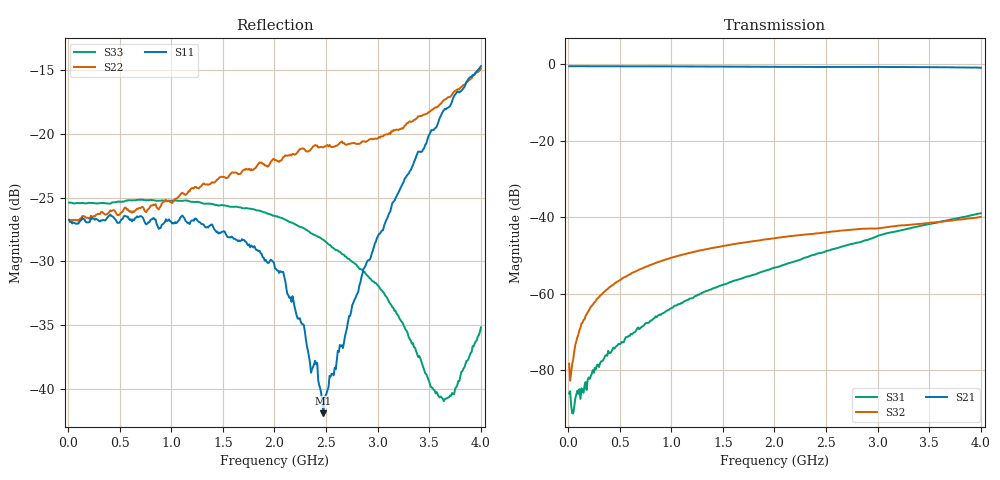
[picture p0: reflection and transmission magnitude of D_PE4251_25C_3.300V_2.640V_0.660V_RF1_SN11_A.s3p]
! Device ID: PE4251_SoldCshunt_081809
! Dir: c:\Test Bench Repositories\Bench_Software_CVI_Version_8\trunk\PSC 4Port_VNA Bench\datalog\4250\TEST\PE4251_SoldCshunt_081809\25C\3p300000\RF1
! Serial: 11
! Insertion: A
! Temp: 25C
! VDD: 3.300
! Control_Hi: 80.000
! Control_Lo: 20.000
! Logic State: RF1
! Port 1: RFC
! Port 2: RF1
! Port 3: RF2
! V1 = 0.66
! V2 = 2.64
! V3 = 0.66
! IDD: 5.417860e-05
! FILE NAME
! DATE 08/18/09  20:12
! CORRECTED  DATA
#  Hz  S  RI  R  50.00
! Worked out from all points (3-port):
!   401 points, 10 MHz to 4 GHz, reference 50 ohm
!   strongest paths, dB at 10 MHz, 1.008 GHz, 2.005 GHz, 3.002 GHz, 4 GHz:
!     S21: -0.6, -0.6, -0.7, -0.7, -1.0
!     S32: -78.3, -50.6, -45.5, -42.9, -39.9
!     S31: -86.0, -63.7, -53.1, -44.9, -39.0
!   lowest |S11| = -41.9 dB at 2.474 GHz (marker M1), VSWR 1.02, Z = 49.9 - j0.801 ohm
!   |S11| at or under -10 dB: start of sweep to end of sweep
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1e7  0.0459 -9e-05  0.9376 -0.00428  5.35e-05 -8.21e-05
     0.9381 -0.00376  0.046 7.23e-05  0.000113 -3.57e-05
     -2.17e-05 -4.49e-05  5.98e-05 0.000106  0.0537 -0.000271
1.19725e8  0.0456 0.00052  0.9382 -0.0415  1.97e-05 -4.38e-05
           0.9381 -0.0412  0.0466 0.000551  4.78e-05 0.000354
           2.13e-06 -4.21e-05  4.24e-05 0.000356  0.0534 -0.000869
1.8955e8  0.0449 -0.000107  0.9366 -0.0642  -1.68e-06 -7.4e-05
          0.9359 -0.0646  0.0469 -0.000551  5.57e-05 0.000561
          -9.66e-07 -7.45e-05  5.49e-05 0.000566  0.0534 -0.00127
5.287e8  0.0462 -0.00324  0.9202 -0.1746  -0.000164 -0.000175
         0.9201 -0.1741  0.0494 -0.00213  0.00017 0.00158
         -0.000148 -0.000177  0.000173 0.00159  0.0541 -0.00479
1.0474e9  0.0418 -0.0158  0.8711 -0.3366  -0.000657 -0.000249
          0.8713 -0.3362  0.0536 -0.015  0.000513 0.00304
          -0.00065 -0.000266  0.000501 0.00304  0.0544 -0.00644
2.005e9  0.0267 -0.0129  0.7145 -0.582  -0.0022 -0.000153
         0.715 -0.5818  0.0686 -0.0388  0.00113 0.00519
         -0.0022 -0.000161  0.00111 0.00519  0.0474 -0.00435
2.473825e9  -0.000508 -0.00802  0.6198 -0.6778  -0.00349 -0.00015
            0.6174 -0.6771  0.0629 -0.062  0.00124 0.00613
            -0.00348 -0.000148  0.00126 0.00615  0.0384 -0.000367
2.8828e9  -0.0211 -0.022  0.5235 -0.7541  -0.00499 7.26e-05
          0.5257 -0.7534  0.041 -0.0832  0.00129 0.00693
          -0.00498 6.37e-05  0.00131 0.00694  0.0282 0.00236
3.62095e9  -0.1003 -0.0656  0.309 -0.8553  -0.00859 0.00175
           0.3104 -0.8561  -0.0476 -0.1236  0.000388 0.00872
           -0.00861 0.00173  0.00039 0.00872  0.00221 0.00898
4e9  -0.1656 -0.0798  0.1755 -0.8804  -0.0108 0.00316
     0.175 -0.8782  -0.1276 -0.1264  -0.000295 0.0101
     -0.0108 0.00315  -0.000321 0.0101  -0.0139 0.0105
